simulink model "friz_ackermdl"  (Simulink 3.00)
settings: Solver=ode45  StartTime=0.0  StopTime=10.0  RelTol=1e-5
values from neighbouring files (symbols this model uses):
  A = 1    [friz_poli.m]    (also in friz_acker.m)
  Fref = 100    [friz_acker.m]
  G0 = MC*inv(-(MA-MB*Kr))*MB    [friz_acker.m]
  Kr = [0 0 1]*inv(Rpiu)*(MA-p_des*eye(3))*(MA-2*p_des*eye(3))*(MA-4*p_des*eye(3))    [friz_acker.m]
  Kv = a    (= 1)    [friz_poli.m]    (also in friz_acker.m)
  P10 = 0    [friz_poli.m]    (also in friz_acker.m)
  x0 = 0    [friz_poli.m]    (also in friz_acker.m)
undefined symbols (not defined in the file or in its folder): b, Cm, Km, mp
libraries: simulink3 x1

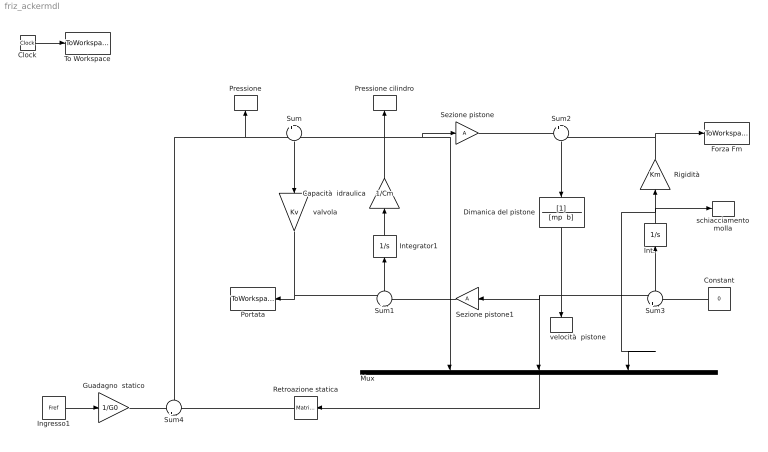
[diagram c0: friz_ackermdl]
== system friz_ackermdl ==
  Capacità  idraulica : Gain  Orientation=up  Gain=1/Cm  SaturateOnIntegerOverflow=on
  Clock : Clock
  Constant : Constant  Orientation=left  Value=0
  Dimanica del pistone : TransferFcn  Orientation=down  Numerator=[1]  Denominator="[mp  b]"
  Forza Fm : ToWorkspace  VariableName=Fm  SampleTime=-1  SaveFormat=Matrix
  Guadagno  statico : Gain  Gain=1/G0  SaturateOnIntegerOverflow=on
  Ingresso1 : Constant  Value=Fref
  Int. : Integrator  Orientation=up  ExternalReset=none  InitialConditionSource=internal  InitialCondition=x0  LimitOutput=off  UpperSaturationLimit=inf  LowerSaturationLimit=-inf  ShowSaturationPort=off  ShowStatePort=off  AbsoluteTolerance=auto
  Integrator1 : Integrator  Orientation=up  ExternalReset=none  InitialConditionSource=internal  InitialCondition=P10  LimitOutput=off  UpperSaturationLimit=inf  LowerSaturationLimit=-inf  ShowSaturationPort=off  ShowStatePort=off  AbsoluteTolerance=auto
  Mux : Mux  Orientation=down  Inputs=3
  Portata : ToWorkspace  VariableName=Q  SampleTime=-1  SaveFormat=Matrix
  Pressione : ToWorkspace  VariableName=P  SampleTime=-1  SaveFormat=Matrix
  Pressione cilindro : ToWorkspace  VariableName=P1  SampleTime=-1  SaveFormat=Matrix
  Retroazione statica : simulink3/Math/Matrix Gain  Orientation=left  K=Kr
  Rigidità : Gain  Orientation=up  Gain=Km  SaturateOnIntegerOverflow=on
  Sezione pistone : Gain  Gain=A  SaturateOnIntegerOverflow=on
  Sezione pistone1 : Gain  Orientation=left  Gain=A  SaturateOnIntegerOverflow=on
  Sum : Sum  Orientation=down  Inputs=+-  SaturateOnIntegerOverflow=on
  Sum1 : Sum  Orientation=up  Inputs=+-  SaturateOnIntegerOverflow=on
  Sum2 : Sum  Orientation=down  Inputs=+-  SaturateOnIntegerOverflow=on
  Sum3 : Sum  Orientation=up  Inputs=+-  SaturateOnIntegerOverflow=on
  Sum4 : Sum  Orientation=up  Inputs=+-  SaturateOnIntegerOverflow=on
  To Workspace : ToWorkspace  VariableName=t  SampleTime=-1  SaveFormat=Matrix
  schiacciamento molla : ToWorkspace  VariableName=x  SampleTime=-1  SaveFormat=Matrix
  valvola : Gain  Orientation=down  Gain=Kv  SaturateOnIntegerOverflow=on
  velocità  pistone : ToWorkspace  VariableName=xdot  SampleTime=-1  SaveFormat=Matrix
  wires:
  Clock/1 -> To Workspace/1
  Int./1 -> Rigidità/1, schiacciamento molla/1, Mux/3
  Sum3/1 -> Int./1
  Rigidità/1 -> Sum2/2, Forza Fm/1
  Constant/1 -> Sum3/2
  Sum2/1 -> Dimanica del pistone/1
  Dimanica del pistone/1 -> Sum3/1, velocità  pistone/1, Sezione pistone1/1, Mux/2
  Sezione pistone/1 -> Sum2/1
  Sum1/1 -> Integrator1/1
  Sezione pistone1/1 -> Sum1/2
  Capacità  idraulica/1 -> Sum/2, Pressione cilindro/1, Sezione pistone/1, Mux/1
  Integrator1/1 -> Capacità  idraulica/1
  Sum/1 -> valvola/1
  valvola/1 -> Portata/1, Sum1/1
  Mux/1 -> Retroazione statica/1
  Retroazione statica/1 -> Sum4/2
  Sum4/1 -> Sum/1, Pressione/1
  Ingresso1/1 -> Guadagno  statico/1
  Guadagno  statico/1 -> Sum4/1
